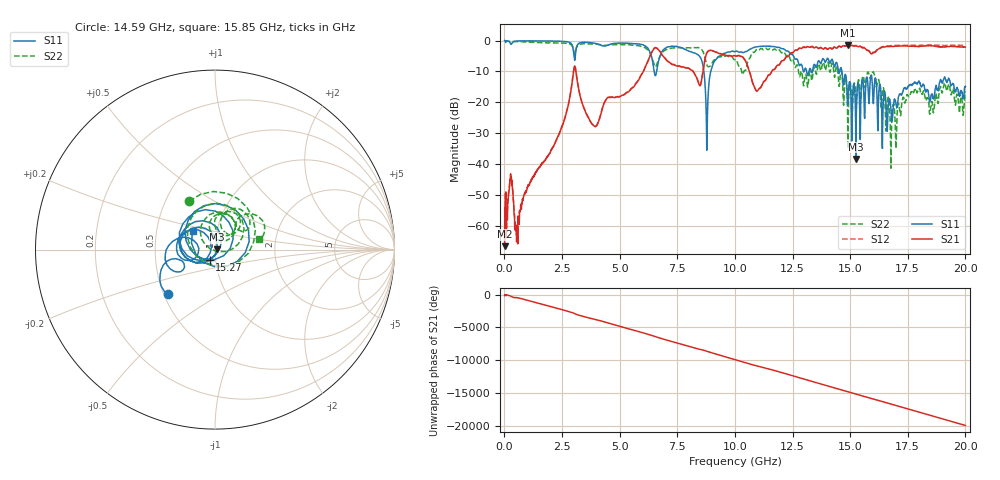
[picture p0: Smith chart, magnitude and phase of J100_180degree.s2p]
!Keysight Technologies,N5222A,MY51421036,A.10.65.16
!Date: Friday, March 31, 2023 14:45:54
!Correction: S11(Full 2 Port(1,2))
!S21(Full 2 Port(1,2))
!S12(Full 2 Port(1,2))
!S22(Full 2 Port(1,2))
!S2P File: Measurements: S11, S21, S12, S22:
# Hz S  dB  R 50
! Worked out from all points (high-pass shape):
!   2000 points, 10 MHz to 20 GHz, reference 50 ohm
!   highest |S21| = -1.58 dB at 14.9 GHz (marker M1); lowest = -66.6 dB at 10 MHz (marker M2)
!   |S21| within 3 dB of the highest: 8.754 GHz to 9.452 GHz (697.9 MHz wide, 7.67 % of centre); 12.37 GHz to end of sweep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
!   lowest |S11| = -38.3 dB at 15.25 GHz (marker M3), VSWR 1.02, Z = 51.2 + j0.219 ohm
!   |S11| at or under -10 dB: 6.499 GHz to 6.603 GHz (104.4 MHz wide, 1.59 % of centre); 8.655 GHz to 8.955 GHz (300.6 MHz wide, 3.41 % of centre); 14.64 GHz to end of sweep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
!   |S22| runs from -41.4 to -0.1 dB; largest |S21 - S12| = 0.066
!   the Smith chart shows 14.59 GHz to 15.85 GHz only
!   S11 on the Smith chart (normalised r, x): 14.59 GHz: 0.53, -0.30; 15.27 GHz: 0.94, -0.11; 15.85 GHz: 0.76, +0.16
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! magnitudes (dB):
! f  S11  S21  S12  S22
! 10 MHz  0.0  -66.6  -64.5  -0.1
! 260 MHz  -0.9  -45.0  -44.5  -0.2
! 550 MHz  -0.1  -60.6  -61.2  -0.3
! 2.47 GHz  -0.3  -28.4  -28.4  -0.8
! 3.03 GHz  -5.7  -8.5  -8.5  -4.2
! 3.35 GHz  -0.7  -19.8  -19.7  -1.1
! 3.97 GHz  -1.0  -27.8  -27.7  -1.2
! 6.68 GHz  -6.9  -2.9  -2.9  -6.3
! 8.39 GHz  -4.6  -13.0  -13.0  -2.3
! 8.79 GHz  -33.6  -3.9  -3.9  -8.0
! 9.11 GHz  -6.8  -3.6  -3.5  -6.3
! 10.01 GHz  -3.6  -4.9  -4.9  -6.2
! 10.98 GHz  -2.0  -16.3  -16.3  -3.0
! 13.34 GHz  -10.4  -1.9  -1.9  -13.0
! 14.59 GHz  -8.8  -2.1  -2.0  -10.3
! 14.9 GHz  -20.5  -1.6  -1.5  -35.0
! 15.25 GHz  -38.3  -1.7  -1.6  -19.6
! 15.27 GHz  -23.6  -1.8  -1.6  -20.8
! 15.85 GHz  -15.8  -3.8  -3.6  -12.0
! 16.67 GHz  -20.1  -2.0  -1.7  -18.5
! 17.88 GHz  -13.9  -1.8  -1.5  -16.2
! 20 GHz  -14.9  -2.1  -1.6  -16.4
